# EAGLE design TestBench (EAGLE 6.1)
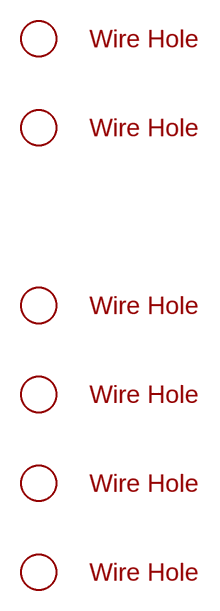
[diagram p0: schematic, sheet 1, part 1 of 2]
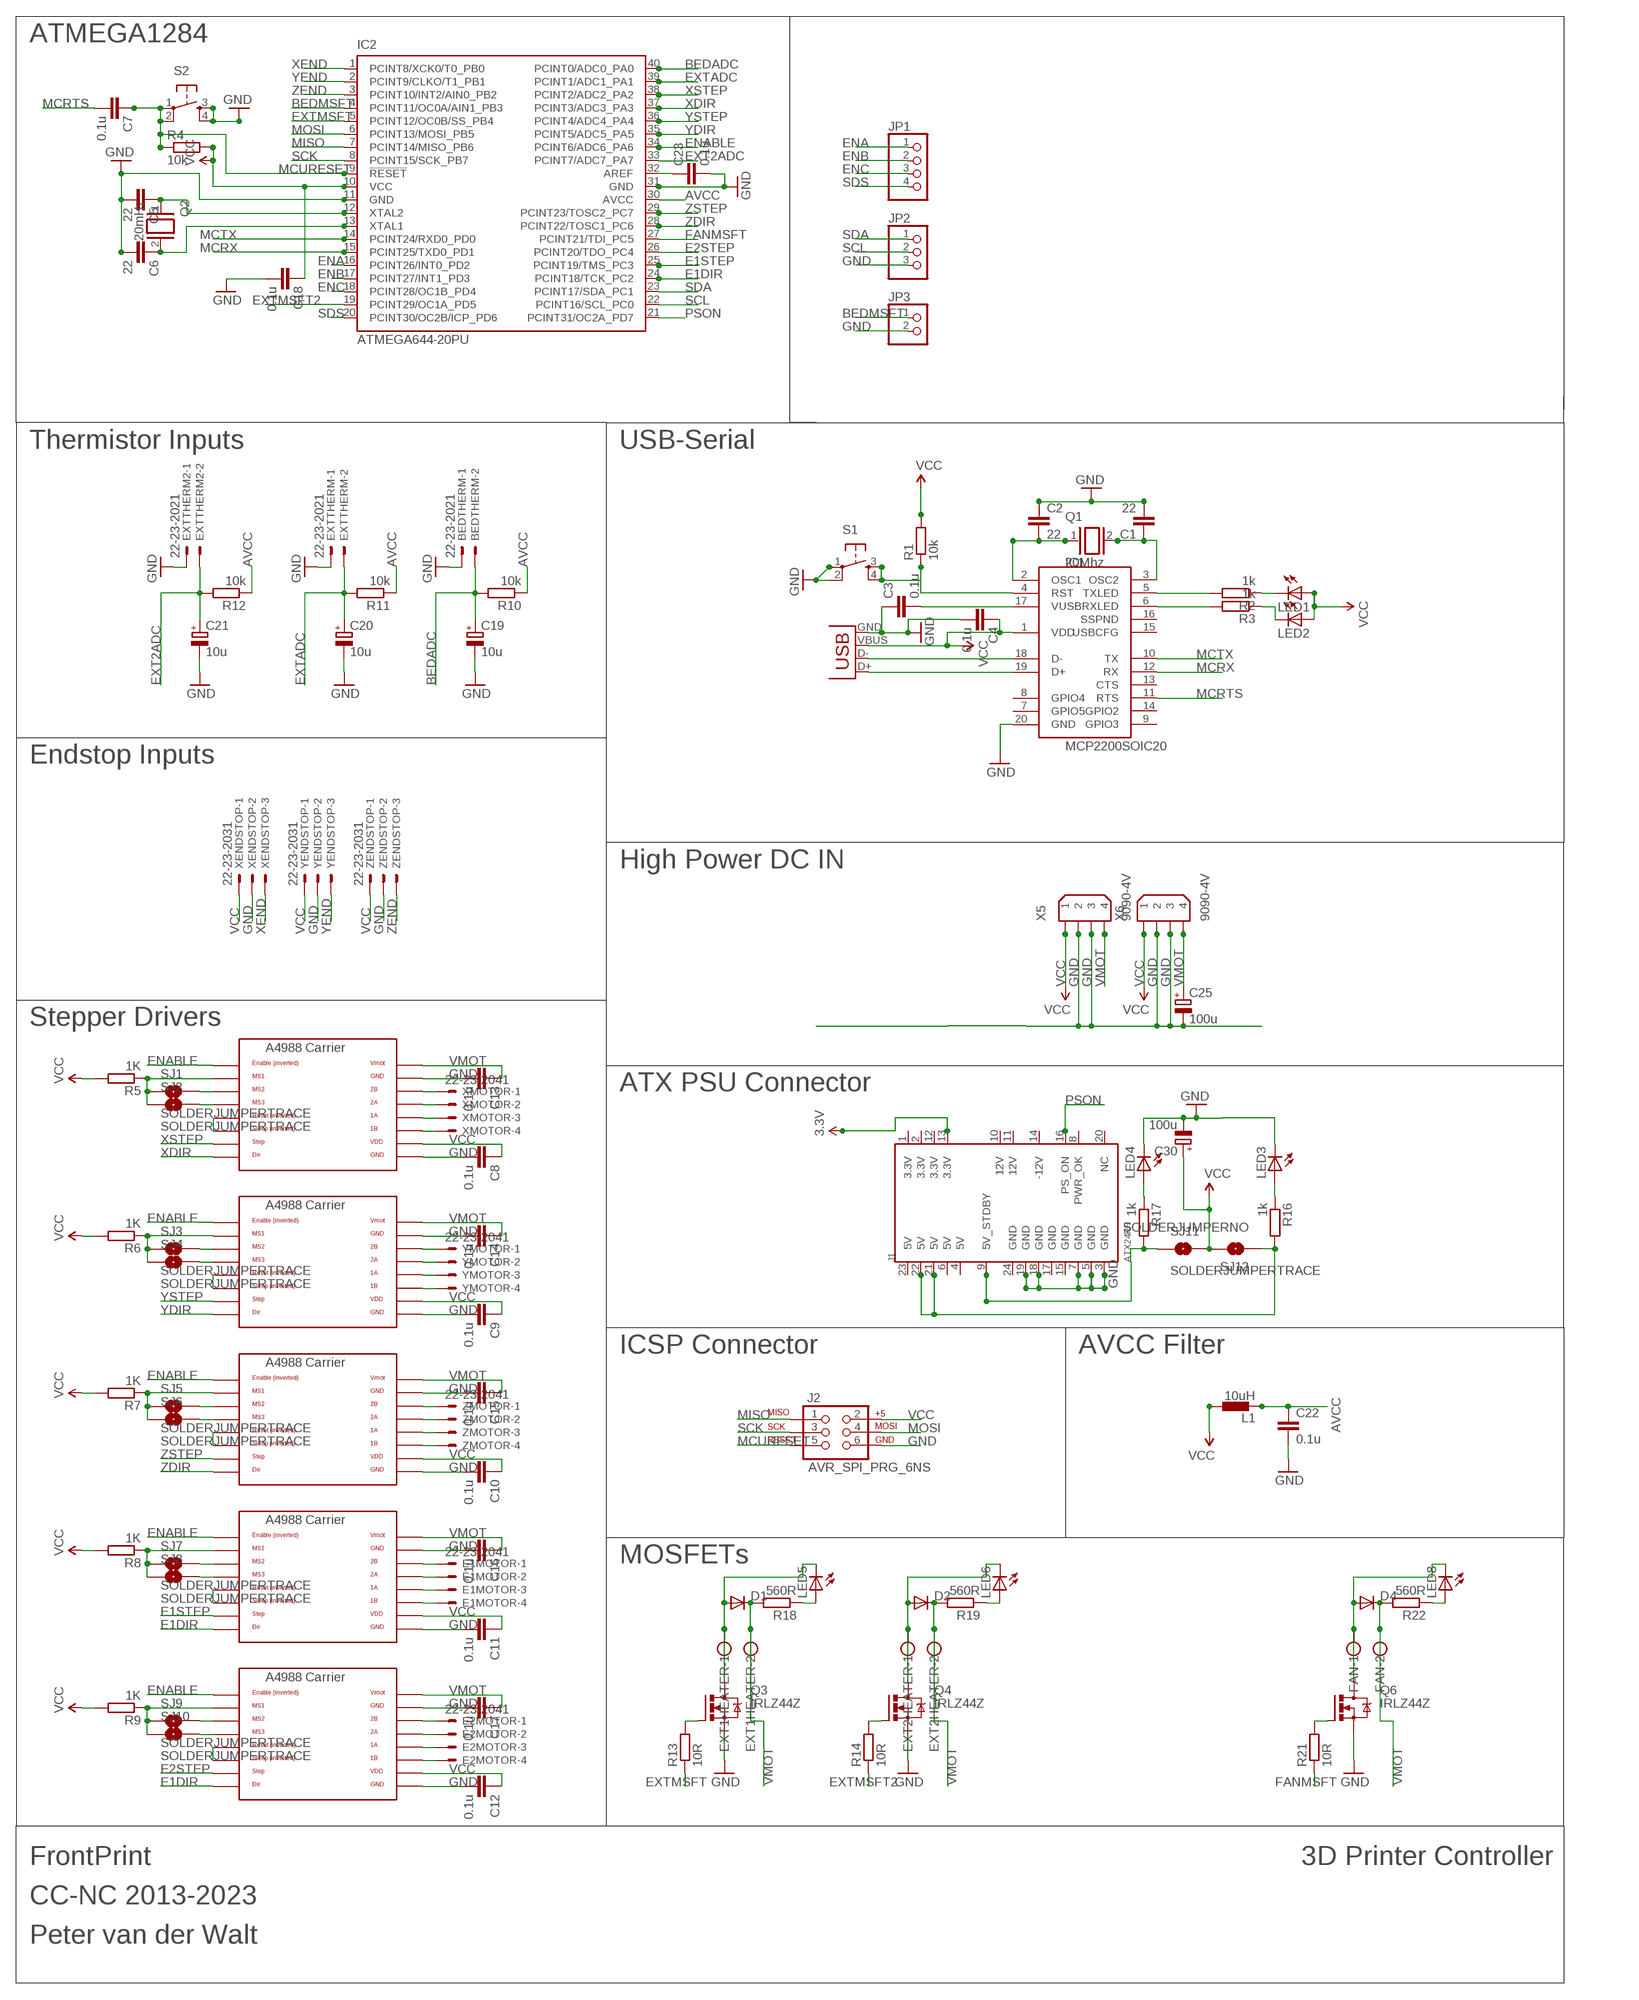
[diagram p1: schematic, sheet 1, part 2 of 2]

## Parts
BEDTHERM  22-23-2021  [22-23-2021]
C1  22  CAPKIT  [CAP-PTH-SMALL-KIT]
C2  22  CAPKIT  [CAP-PTH-SMALL-KIT]
C3  0.1u  CAPKIT  [CAP-PTH-SMALL-KIT]
C4  0.1u  CAPKIT  [CAP-PTH-SMALL-KIT]
C5  22  CAPKIT  [CAP-PTH-SMALL-KIT]
C6  22  CAPKIT  [CAP-PTH-SMALL-KIT]
C7  0.1u  CAPKIT  [CAP-PTH-SMALL-KIT]
C8  0.1u  CAPKIT  [CAP-PTH-SMALL-KIT]
C9  0.1u  CAPKIT  [CAP-PTH-SMALL-KIT]
C10  0.1u  CAPKIT  [CAP-PTH-SMALL-KIT]
C11  0.1u  CAPKIT  [CAP-PTH-SMALL-KIT]
C12  0.1u  CAPKIT  [CAP-PTH-SMALL-KIT]
C13  0.1u  CAPKIT  [CAP-PTH-SMALL-KIT]
C14  0.1u  CAPKIT  [CAP-PTH-SMALL-KIT]
C15  0.1u  CAPKIT  [CAP-PTH-SMALL-KIT]
C16  0.1u  CAPKIT  [CAP-PTH-SMALL-KIT]
C17  0.1u  CAPKIT  [CAP-PTH-SMALL-KIT]
C18  0.1u  CAPKIT  [CAP-PTH-SMALL-KIT]
C19  10u  CPOL-EUE2.5-5  [E2,5-5]
C20  10u  CPOL-EUE2.5-5  [E2,5-5]
C21  10u  CPOL-EUE2.5-5  [E2,5-5]
C22  0.1u  CAPKIT  [CAP-PTH-SMALL-KIT]
C23  0.1u  CAPKIT  [CAP-PTH-SMALL-KIT]
C25  100u  CPOL-EUE5-8.5  [E5-8,5]
C30  100u  CPOL-EUE5-8.5  [E5-8,5]
D1  DIODE1N4148  [DIODE-1N4148]
D2  DIODE1N4148  [DIODE-1N4148]
D4  DIODE1N4148  [DIODE-1N4148]
E1MOTOR  22-23-2041  [22-23-2041]
E2MOTOR  22-23-2041  [22-23-2041]
EPOLOLU  POLOLU_A4983CARRIER  [A4988BREAKOUT]
EPOLOLU2  POLOLU_A4983CARRIER  [A4988BREAKOUT]
EXT1HEATER  W237-102  [W237-102]
EXT2HEATER  W237-102  [W237-102]
EXTTHERM  22-23-2021  [22-23-2021]
EXTTHERM2  22-23-2021  [22-23-2021]
FAN  W237-102  [W237-102]
IC1  MCP2200SOIC20  [SOIC20]
IC2  ATMEGA644-20PU  [DIL40]
J1  ATX24RH  [ATX24_RIGHT_ANGLE]
J2  AVR_SPI_PRG_6NS  [2X3-NS]
JP1  PINHD-1X4  [1X04]
JP2  PINHD-1X3  [1X03]
JP3  PINHD-1X2  [1X02]
L1  10uH  BL01RN1A  [BL01RN1A]
LED1  LED3MM  [LED3MM]
LED2  LED3MM  [LED3MM]
LED3  LED3MM  [LED3MM]
LED4  LED3MM  [LED3MM]
LED5  LED3MM  [LED3MM]
LED6  LED3MM  [LED3MM]
LED8  LED3MM  [LED3MM]
Q1  20Mhz  XTAL/S  [QS]
Q2  20mHz  XTAL/S  [QS]
Q3  IRLZ44Z  [TO220BH]
Q4  IRLZ44Z  [TO220BH]
Q6  IRLZ44Z  [TO220BH]
R1  10k  R-EU_0204/7  [0204/7]
R2  1k  R-EU_0204/7  [0204/7]
R3  1k  R-EU_0204/7  [0204/7]
R4  10k  R-EU_0204/7  [0204/7]
R5  1K  R-EU_0204/7  [0204/7]
R6  1K  R-EU_0204/7  [0204/7]
R7  1K  R-EU_0204/7  [0204/7]
R8  1K  R-EU_0204/7  [0204/7]
R9  1K  R-EU_0204/7  [0204/7]
R10  10k  R-EU_0204/7  [0204/7]
R11  10k  R-EU_0204/7  [0204/7]
R12  10k  R-EU_0204/7  [0204/7]
R13  10R  R-EU_0204/7  [0204/7]
R14  10R  R-EU_0204/7  [0204/7]
R16  1k  R-EU_0204/7  [0204/7]
R17  1k  R-EU_0204/7  [0204/7]
R18  560R  R-EU_0204/7  [0204/7]
R19  560R  R-EU_0204/7  [0204/7]
R21  10R  R-EU_0204/7  [0204/7]
R22  560R  R-EU_0204/7  [0204/7]
S1  TAC_SWITCHPTH  [TACTILE-PTH]
S2  TAC_SWITCHPTH  [TACTILE-PTH]
SJ1  SOLDERJUMPERTRACE  [SJ_2S-TRACE]
SJ2  SOLDERJUMPERTRACE  [SJ_2S-TRACE]
SJ3  SOLDERJUMPERTRACE  [SJ_2S-TRACE]
SJ4  SOLDERJUMPERTRACE  [SJ_2S-TRACE]
SJ5  SOLDERJUMPERTRACE  [SJ_2S-TRACE]
SJ6  SOLDERJUMPERTRACE  [SJ_2S-TRACE]
SJ7  SOLDERJUMPERTRACE  [SJ_2S-TRACE]
SJ8  SOLDERJUMPERTRACE  [SJ_2S-TRACE]
SJ9  SOLDERJUMPERTRACE  [SJ_2S-TRACE]
SJ10  SOLDERJUMPERTRACE  [SJ_2S-TRACE]
SJ11  SOLDERJUMPERTRACE  [SJ_2S-TRACE]
SJ12  SOLDERJUMPERNO  [SJ_2S-NO]
U$1  3MMHOLE  [3MMHOLE]
U$3  3MMHOLE  [3MMHOLE]
U$5  3MMHOLE  [3MMHOLE]
U$6  3MMHOLE  [3MMHOLE]
U$7  3MMHOLE  [3MMHOLE]
U$8  3MMHOLE  [3MMHOLE]
X1  USBPTH  [USB-B-PTH]
X5  9090-4V  [9090-4V]
X6  9090-4V  [9090-4V]
XENDSTOP  22-23-2031  [22-23-2031]
XMOTOR  22-23-2041  [22-23-2041]
XPOLOLU  POLOLU_A4983CARRIER  [A4988BREAKOUT]
YENDSTOP  22-23-2031  [22-23-2031]
YMOTOR  22-23-2041  [22-23-2041]
YPOLOLU  POLOLU_A4983CARRIER  [A4988BREAKOUT]
ZENDSTOP  22-23-2031  [22-23-2031]
ZMOTOR  22-23-2041  [22-23-2041]
ZPOLOLU  POLOLU_A4983CARRIER  [A4988BREAKOUT]

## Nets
3.3V: J1.13(3.3V)
AVCC: C22.1 IC2.30(AVCC) L1.1 R10.1 R11.1 R12.1
BEDADC: BEDTHERM.2 C19.+ IC2.40(PCINT0/ADC0_PA0) R10.2
BEDMSFT: IC2.4(PCINT11/OC0A/AIN1_PB3) JP3.1
E1DIR: EPOLOLU2.DIR EPOLOLU.DIR IC2.24(PCINT18/TCK_PC2)
E1STEP: EPOLOLU.STEP IC2.25(PCINT19/TMS_PC3)
E2STEP: EPOLOLU2.STEP IC2.26(PCINT20/TDO_PC4)
ENA: IC2.16(PCINT26/INT0_PD2) JP1.1
ENABLE: EPOLOLU2.EN EPOLOLU.EN IC2.34(PCINT6/ADC6_PA6) XPOLOLU.EN YPOLOLU.EN ZPOLOLU.EN
ENB: IC2.17(PCINT27/INT1_PD3) JP1.2
ENC: IC2.18(PCINT28/OC1B_PD4) JP1.3
EXT2ADC: C21.+ EXTTHERM2.2 IC2.33(PCINT7/ADC7_PA7) R12.2
EXTADC: C20.+ EXTTHERM.2 IC2.39(PCINT1/ADC1_PA1) R11.2
EXTMSFT: IC2.5(PCINT12/OC0B/SS_PB4) R13.1
EXTMSFT2: IC2.19(PCINT29/OC1A_PD5) R14.1
FANMSFT: IC2.27(PCINT21/TDI_PC5) R21.1
GND: BEDTHERM.1 C1.2 C2.1 C3.1 C4.2 C5.2 C6.2 C8.2 C9.2 C10.2 C11.2 C12.2 C13.2 C14.2 C15.2 C16.2 C17.2 C18.2 C19.- C20.- C21.- C22.2 C23.2 C25.- C30.- EPOLOLU2.GND EPOLOLU2.GND@0(GND) EPOLOLU.GND EPOLOLU.GND@0(GND) EXTTHERM2.1 EXTTHERM.1 IC1.20(GND) IC2.11(GND) IC2.31(GND) J1.3(GND) J1.5(GND) J1.7(GND) J1.18(GND) J1.19(GND) J2.6 JP2.3 JP3.2 LED3.K(C) LED4.K(C) Q3.S Q4.S Q6.S S1.1 S1.2 S2.3 S2.4 X1.GND X5.2 X5.3 X6.2 X6.3 XENDSTOP.2 XPOLOLU.GND XPOLOLU.GND@0(GND) YENDSTOP.2 YPOLOLU.GND YPOLOLU.GND@0(GND) ZENDSTOP.2 ZPOLOLU.GND ZPOLOLU.GND@0(GND)
MCRTS: C7.2 IC1.11(RTS)
MCRX: IC1.12(RX) IC2.15(PCINT25/TXD0_PD1)
MCTX: IC1.10(TX) IC2.14(PCINT24/RXD0_PD0)
MCURESET: C7.1 IC2.9(!RESET) J2.5 R4.1 S2.1 S2.2
MISO: IC2.7(PCINT14/MISO_PB6) J2.1
MOSI: IC2.6(PCINT13/MOSI_PB5) J2.4
N$1: C2.2 IC1.2(OSC1) Q1.1
N$2: C1.1 IC1.3(OSC2) Q1.2
N$3: IC1.5(TXLED) R2.2
N$4: IC1.18(D-) X1.D-
N$5: IC1.19(D+) X1.D+
N$6: IC1.6(RXLED) R3.2
N$7: C3.2 IC1.17(VUSB)
N$8: Q3.G R13.2
N$9: LED1.K(C) R2.1
N$10: LED2.K(C) R3.1
N$11: C5.1 IC2.12(XTAL2) Q2.1
N$12: C6.1 IC2.13(XTAL1) Q2.2
N$13: IC1.4(RST) R1.1 S1.3 S1.4
N$14: R7.1 SJ5.1 SJ6.1 ZPOLOLU.MS1
N$15: SJ6.2 ZPOLOLU.MS3
N$16: SJ5.2 ZPOLOLU.MS2
N$17: EPOLOLU.MS2 SJ7.2
N$18: EPOLOLU.MS3 SJ8.2
N$19: EPOLOLU.MS1 R8.1 SJ7.1 SJ8.1
N$20: SJ3.2 YPOLOLU.MS2
N$21: SJ4.2 YPOLOLU.MS3
N$22: R6.1 SJ3.1 SJ4.1 YPOLOLU.MS1
N$23: SJ1.2 XPOLOLU.MS2
N$24: SJ2.2 XPOLOLU.MS3
N$25: R5.1 SJ1.1 SJ2.1 XPOLOLU.MS1
N$26: XPOLOLU.RST XPOLOLU.SLP(SLEEP)
N$27: YPOLOLU.RST YPOLOLU.SLP(SLEEP)
N$28: ZPOLOLU.RST ZPOLOLU.SLP(SLEEP)
N$29: EPOLOLU.RST EPOLOLU.SLP(SLEEP)
N$30: E1MOTOR.1 EPOLOLU.2B
N$31: E1MOTOR.2 EPOLOLU.2A
N$32: E1MOTOR.3 EPOLOLU.1A
N$33: E1MOTOR.4 EPOLOLU.1B
N$34: ZMOTOR.4 ZPOLOLU.1B
N$35: ZMOTOR.3 ZPOLOLU.1A
N$36: ZMOTOR.2 ZPOLOLU.2A
N$37: ZMOTOR.1 ZPOLOLU.2B
N$38: YMOTOR.4 YPOLOLU.1B
N$39: YMOTOR.3 YPOLOLU.1A
N$40: YMOTOR.2 YPOLOLU.2A
N$41: YMOTOR.1 YPOLOLU.2B
N$42: XMOTOR.4 XPOLOLU.1B
N$43: XMOTOR.3 XPOLOLU.1A
N$44: XMOTOR.2 XPOLOLU.2A
N$45: XMOTOR.1 XPOLOLU.2B
N$46: EPOLOLU2.MS2 SJ9.2
N$47: EPOLOLU2.MS3 SJ10.2
N$48: EPOLOLU2.MS1 R9.1 SJ9.1 SJ10.1
N$49: EPOLOLU2.RST EPOLOLU2.SLP(SLEEP)
N$50: E2MOTOR.1 EPOLOLU2.2B
N$51: E2MOTOR.2 EPOLOLU2.2A
N$52: E2MOTOR.3 EPOLOLU2.1A
N$53: E2MOTOR.4 EPOLOLU2.1B
N$54: C23.1 IC2.32(AREF)
N$55: D1.A EXT1HEATER.1 LED5.K(C) Q3.D
N$56: Q4.G R14.2
N$57: D2.A EXT2HEATER.1 LED6.K(C) Q4.D
N$60: J1.21(5V) J1.22(5V) R16.2 SJ12.1
N$61: LED5.A R18.1
N$62: J1.9(5V_STDBY) R17.2 SJ11.1
N$63: LED4.A R17.1
N$64: LED3.A R16.1
N$65: Q6.G R21.2
N$66: LED6.A R19.1
N$67: D4.A FAN.1 LED8.K(C) Q6.D
N$69: LED8.A R22.1
PSON: IC2.21(PCINT31/OC2A_PD7) J1.16(PS_ON)
SCK: IC2.8(PCINT15/SCK_PB7) J2.3
SCL: IC2.22(PCINT16/SCL_PC0) JP2.2
SDA: IC2.23(PCINT17/SDA_PC1) JP2.1
SDS: IC2.20(PCINT30/OC2B/ICP_PD6) JP1.4
VCC: C4.1 C8.1 C9.1 C10.1 C11.1 C12.1 C18.1 C30.+ EPOLOLU2.VDD EPOLOLU.VDD IC1.1(VDD) IC2.10(VCC) J2.2 L1.2 LED1.A LED2.A R1.2 R4.2 R5.2 R6.2 R7.2 R8.2 R9.2 SJ11.2 SJ12.2 X1.VBUS X5.1 X6.1 XENDSTOP.1 XPOLOLU.VDD YENDSTOP.1 YPOLOLU.VDD ZENDSTOP.1 ZPOLOLU.VDD
VMOT: C13.1 C14.1 C15.1 C16.1 C17.1 C25.+ D1.C D2.C D4.C EPOLOLU2.VMOT EPOLOLU.VMOT EXT1HEATER.2 EXT2HEATER.2 FAN.2 R18.2 R19.2 R22.2 X5.4 X6.4 XPOLOLU.VMOT YPOLOLU.VMOT ZPOLOLU.VMOT
XDIR: IC2.37(PCINT3/ADC3_PA3) XPOLOLU.DIR
XEND: IC2.1(PCINT8/XCK0/T0_PB0) XENDSTOP.3
XSTEP: IC2.38(PCINT2/ADC2_PA2) XPOLOLU.STEP
YDIR: IC2.35(PCINT5/ADC5_PA5) YPOLOLU.DIR
YEND: IC2.2(PCINT9/CLKO/T1_PB1) YENDSTOP.3
YSTEP: IC2.36(PCINT4/ADC4_PA4) YPOLOLU.STEP
ZDIR: IC2.28(PCINT22/TOSC1_PC6) ZPOLOLU.DIR
ZEND: IC2.3(PCINT10/INT2/AIN0_PB2) ZENDSTOP.3
ZSTEP: IC2.29(PCINT23/TOSC2_PC7) ZPOLOLU.STEP
Unconnected: IC1.7(GPIO5) IC1.8(GPIO4) IC1.9(GPIO3) IC1.13(CTS) IC1.14(GPIO2) IC1.15(USBCFG) IC1.16(SSPND) J1.1(3.3V) J1.2(3.3V) J1.4(5V) J1.6(5V) J1.8(PWR_OK) J1.10(12V) J1.11(12V) J1.12(3.3V) J1.14(-12V) J1.15(GND) J1.17(GND) J1.20(NC) J1.23(5V) J1.24(GND)

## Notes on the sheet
- ATMEGA1284
- Thermistor Inputs | USB-Serial
- Endstop Inputs
- High Power DC IN
- Stepper Drivers
- ATX PSU Connector
- ICSP Connector | AVCC Filter
- MOSFETs
- FrontPrint | 3D Printer Controller
- CC-NC 2013-2023
- Peter van der Walt

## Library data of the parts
BEDTHERM EXTTHERM EXTTHERM2 = con-molex:22-23-2021: .100" (2.54mm) Center Header - 2 Pin; MF: MOLEX; MPN: 22-23-2021; OC_FARNELL: 1462926; OC_NEWARK: 25C3832
C1-C18 C22 C23 = SparkFun-Passives:CAP: Capacitor
C19-C21 C25 C30 = rcl:CPOL-EU: POLARIZED CAPACITOR, European symbol
D1 D2 D4 = SparkFun-DiscreteSemi:DIODE: Diode
E1MOTOR E2MOTOR XMOTOR YMOTOR ZMOTOR = con-molex:22-23-2041: .100" (2.54mm) Center Header - 4 Pin; MF: MOLEX; MPN: 22-23-2041; OC_FARNELL: 1462920; OC_NEWARK: 38C0355
EPOLOLU EPOLOLU2 XPOLOLU YPOLOLU ZPOLOLU = RepRapjr:POLOLU_A4983CARRIER
EXT1HEATER EXT2HEATER FAN = con-wago-500:W237-102: WAGO SCREW CLAMP; MPN: 237-102; OC_FARNELL: unknown; OC_NEWARK: 70K9898
IC1 = microchip-update-2:MCP2200: USB 2.0 to UART Protocol Converter with GPIO
IC2 = atmel:ATMEGA644-*PU: 8-bit Microcontroller with 64K Bytes In-System Programmable Flash Auto generated by make-symbol-device-package-bsdl.ulp Rev. 34 Source: http://www.atmel.com/dyn/resources/prod_documents/doc2593.pdf; MPN: ATMEGA644-20PU; OC_FARNELL: 1288340; OC_NEWARK: 23M5060
J1 = SparkFun-Connectors:ATX24: ATX24 Pin Power Supply Connector This is a good connector for connecting a computer power supply to a PCB. It's massive, but provides many amps of power at 5V and 12V. SKU: PRT-09498
J2 = SparkFun-Connectors:AVR_SPI_PRG_6: AVR ISP 6 Pin This is the reduced ISP connector for AVR programming. Common on Arduino. This footprint will take up less PCB space and can be used with a 10-pin to 6-pin adapter such as SKU: BOB-08508
JP1 = pinhead:PINHD-1X4: PIN HEADER
JP2 = pinhead:PINHD-1X3: PIN HEADER
JP3 = pinhead:PINHD-1X2: PIN HEADER
L1 = inductors:BL0: Noise Suppression Products/EMI Suppression Filters, Lead EMIFIL(R) Inductor Type
LED1-LED6 LED8 = led:LED: LED
Q1 Q2 = special:XTAL/S: CRYSTAL
Q3 Q4 Q6 = transistor-power:IRLZ44Z: N-Channel HEXFET® Power MOSFET Logic Level AUTOMOTIVE MOSFET Source: http://www.irf.com/product-info/datasheets/data/irlz44zpbf.pdf
R1-R14 R16-R19 R21 R22 = resistor:R-EU_: RESISTOR, European symbol
S1 S2 = SparkFun-Electromechanical:TAC_SWITCH: Momentary Switch Button commonly used for reset or general input. Spark Fun Electronics SKU : COM-00097
SJ1-SJ12 = SparkFun-Passives:SOLDERJUMPER: Solder Jumper
U$1 U$3 U$5-U$8 = reprap:3MMHOLE
X1 = SparkFun-Connectors:USB: USB Connectors USB-B-PTH is fully proven SKU : PRT-00139 USB-miniB is fully proven SKU : PRT-00587 USB-A-PCB is untested. USB-A-H is throughly reviewed, but untested. Spark Fun Electronics SKU : PRT-00437 USB-B-SMT is throughly reviewed, but untested. Needs silkscreen touching up. USB-A-S has not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
X5 X6 = con-thomas-betts:9090-4: Disk Drive Power four position Source: Thomas & Betts Electronic Interconnects Eiropean Edition 1998; OC_FARNELL: unknown; OC_NEWARK: unknown
XENDSTOP YENDSTOP ZENDSTOP = con-molex:22-23-2031: .100" (2.54mm) Center Header - 3 Pin; MF: MOLEX; MPN: 22-23-2031; OC_FARNELL: 1462950; OC_NEWARK: 30C0862

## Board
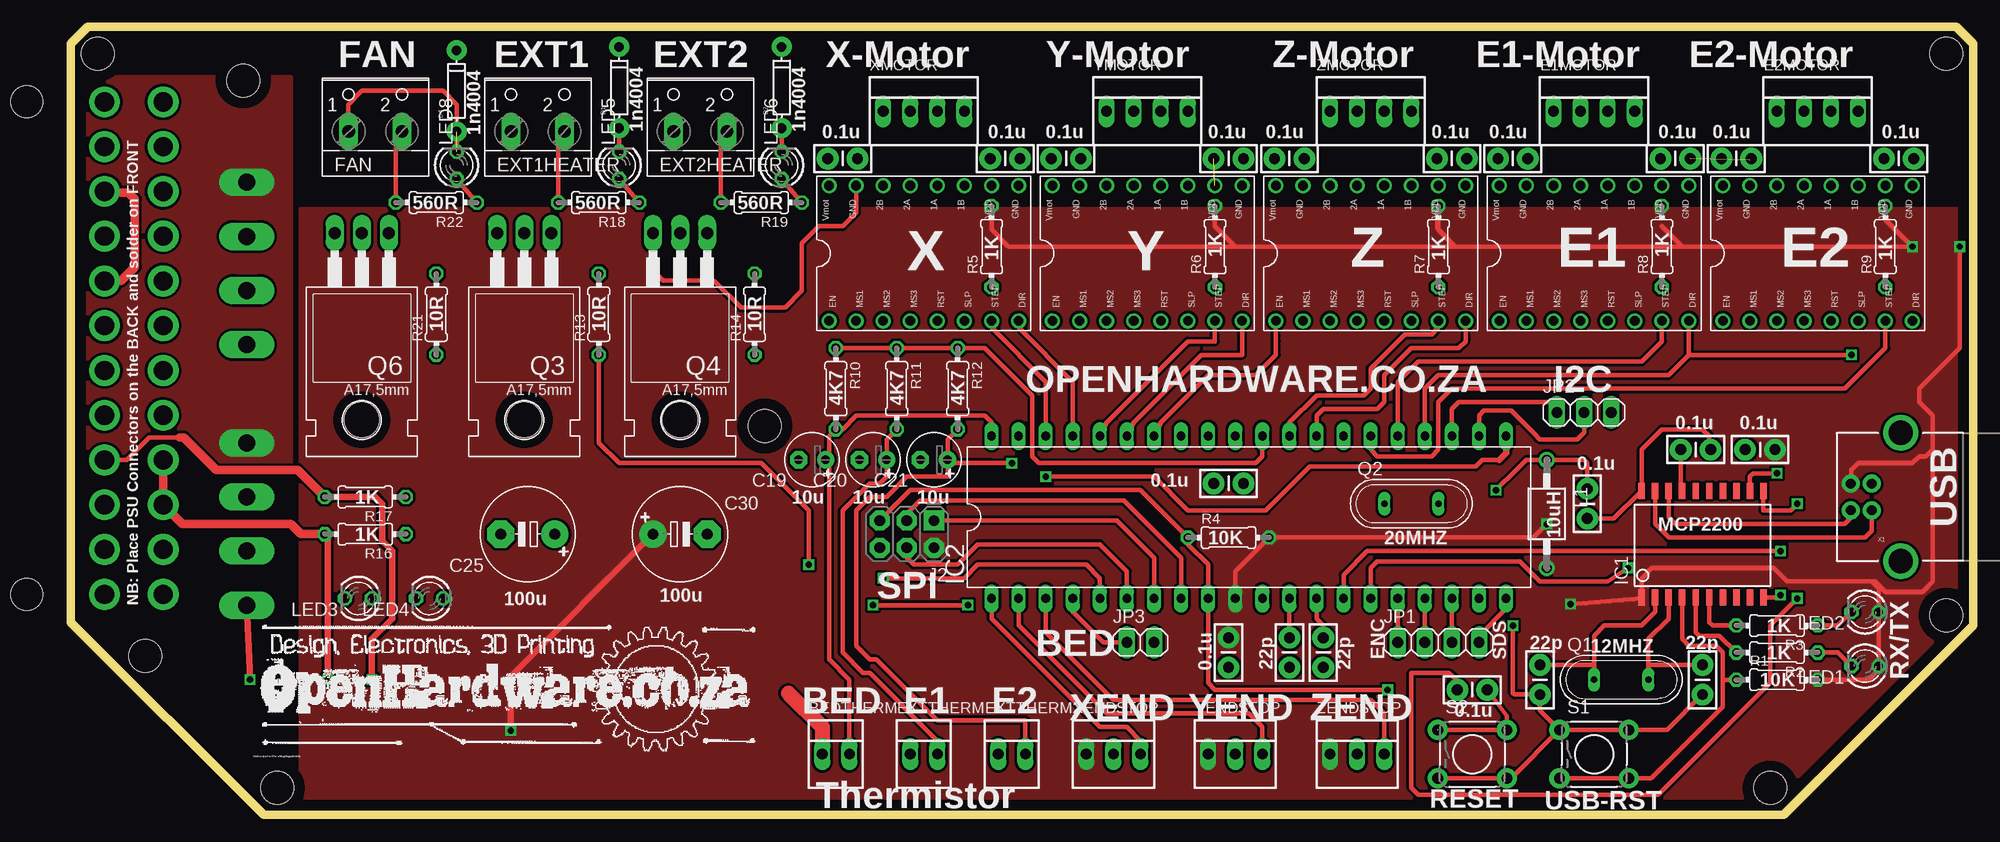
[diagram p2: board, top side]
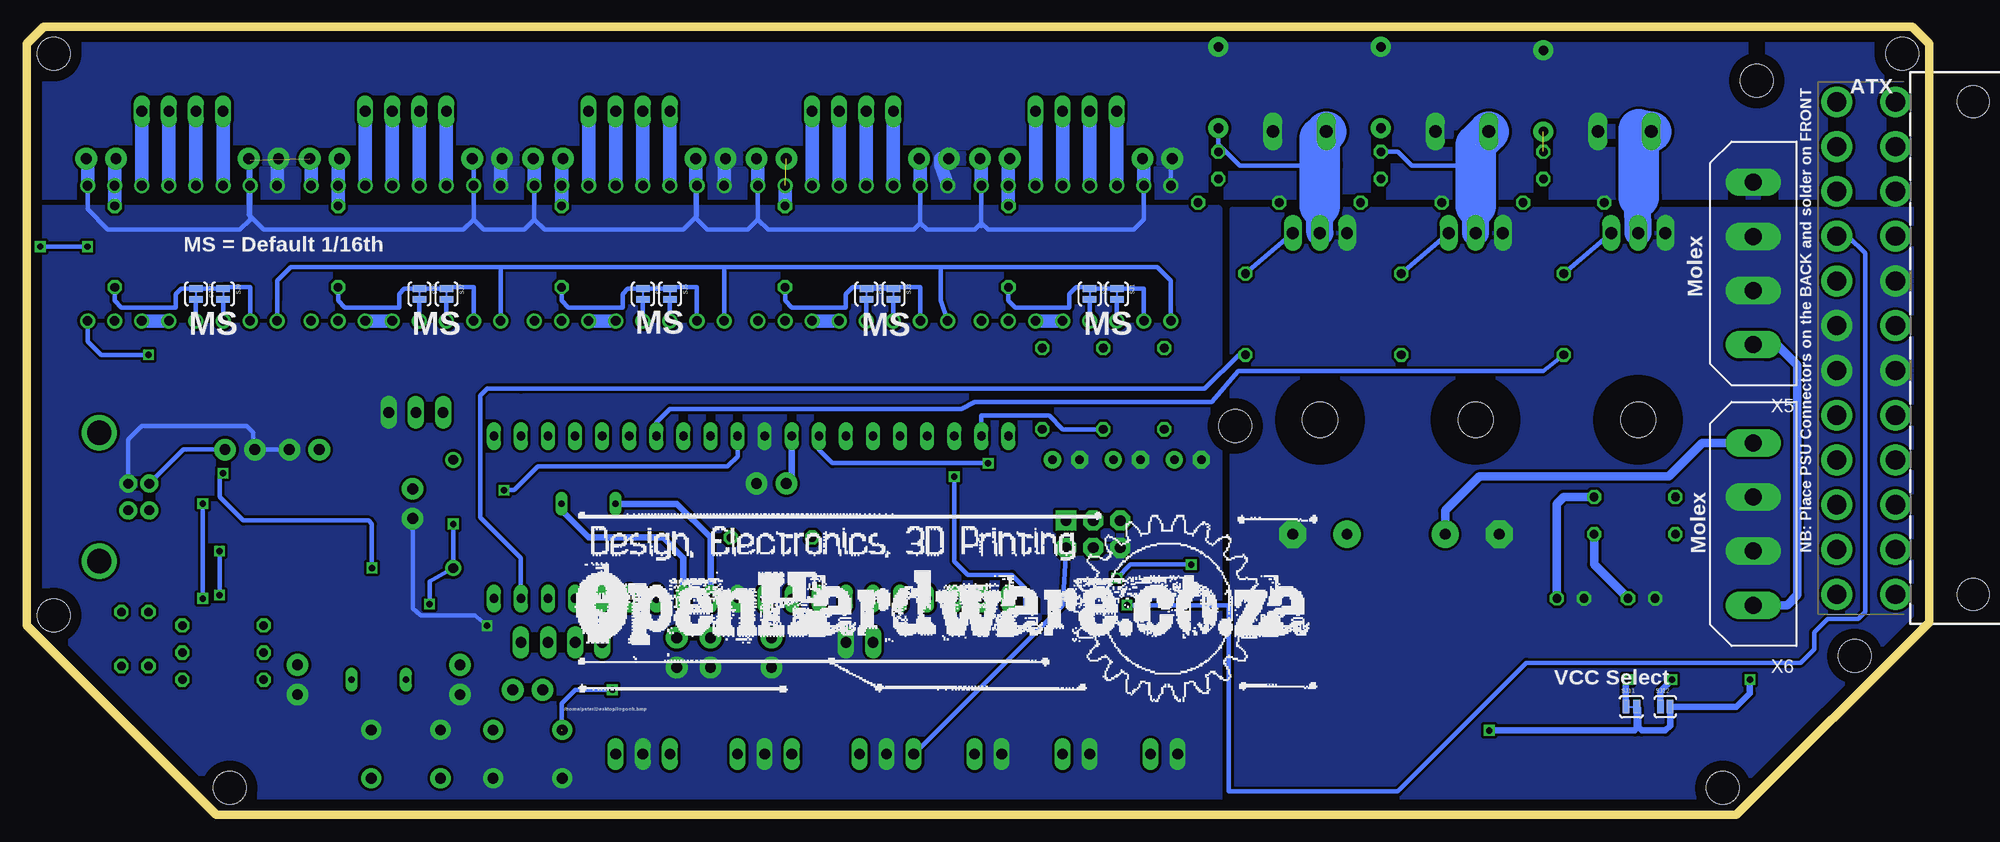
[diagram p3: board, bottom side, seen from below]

Size 178.44 x 73.98 mm. Coordinates in mm from the lower left corner, seen from the top.
Outline: 0,72.39 0,18.1 18.1,0 160.65,0 178.43,17.78 178.43,72.39 176.85,73.98 1.59,73.98 0,72.39
Copper layers (1*16): Top 0.035mm / dielectric 1.5mm / Bottom 0.035mm
Design rules: minimum track width 10mil, minimum drill 20mil, track to track 10mil, track to pad 10mil, pad to pad 10mil, via to via 10mil, smd to smd 10mil, copper to edge 40mil, drill to drill 8mil, minimum pad ring 10mil, minimum via ring 8mil, stop-mask expansion 1mil, vias tented up to drill 0mil, thermal gap 0mil

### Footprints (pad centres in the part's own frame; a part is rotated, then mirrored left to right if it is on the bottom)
22-23-2021 = drill 1 long: 1 -1.27,0; 2 1.27,0
CAP-PTH-SMALL-KIT = drill 1.016 pad 2.032: 1 -1.397,0; 2 1.397,0
E2,5-5 = drill 0.813 pad 1.6: + -1.27,0 | drill 0.813 pad 1.6 octagon: - 1.27,0
E5-8,5 = drill 1.016 pad 2.54: + -2.54,0 | drill 1.016 pad 2.54 octagon: - 2.54,0
DIODE-1N4148 = drill 0.9 pad 1.88: A -3.81,0; C 3.81,0
22-23-2041 = drill 1 long: 1 -3.81,0; 2 -1.27,0; 3 1.27,0; 4 3.81,0
A4988BREAKOUT = drill 0.9: 1A 8.89,1.27; 1B 11.43,1.27; 2A 6.35,1.27; 2B 3.81,1.27; DIR 16.51,-11.43; EN -1.27,-11.43; GND 16.51,1.27; GND@0 1.27,1.27; MS1 1.27,-11.43; MS2 3.81,-11.43; MS3 6.35,-11.43; RST 8.89,-11.43; SLP 11.43,-11.43; STEP 13.97,-11.43; VDD 13.97,1.27; VMOT -1.27,1.27
W237-102 = drill 1.194 long: 1 -2.5,-1.27; 2 2.5,-1.27
SOIC20 = smd 0.6 x 1.5: 1 -5.715,-5; 2 -4.445,-5; 3 -3.175,-5; 4 -1.905,-5; 5 -0.635,-5; 6 0.635,-5; 7 1.905,-5; 8 3.175,-5; 9 4.445,-5; 10 5.715,-5; 11 5.715,5; 12 4.445,5; 13 3.175,5; 14 1.905,5; 15 0.635,5; 16 -0.635,5; 17 -1.905,5; 18 -3.175,5; 19 -4.445,5; 20 -5.715,5
DIL40 = drill 0.813 long: 1 -24.13,-7.62; 2 -21.59,-7.62; 3 -19.05,-7.62; 4 -16.51,-7.62; 5 -13.97,-7.62; 6 -11.43,-7.62; 7 -8.89,-7.62; 8 -6.35,-7.62; 9 -3.81,-7.62; 10 -1.27,-7.62; 11 1.27,-7.62; 12 3.81,-7.62; 13 6.35,-7.62; 14 8.89,-7.62; 15 11.43,-7.62; 16 13.97,-7.62; 17 16.51,-7.62; 18 19.05,-7.62; 19 21.59,-7.62; 20 24.13,-7.62; 21 24.13,7.62; 22 21.59,7.62; 23 19.05,7.62; 24 16.51,7.62; 25 13.97,7.62; 26 11.43,7.62; 27 8.89,7.62; 28 6.35,7.62; 29 3.81,7.62; 30 1.27,7.62; 31 -1.27,7.62; 32 -3.81,7.62; 33 -6.35,7.62; 34 -8.89,7.62; 35 -11.43,7.62; 36 -13.97,7.62; 37 -16.51,7.62; 38 -19.05,7.62; 39 -21.59,7.62; 40 -24.13,7.62
ATX24_RIGHT_ANGLE = drill 1.8 pad 2.9: 1 23.1,4.76; 2 18.9,4.76; 3 14.7,4.76; 4 10.5,4.76; 5 6.3,4.76; 6 2.1,4.76; 7 -2.1,4.76; 8 -6.3,4.76; 9 -10.5,4.76; 10 -14.7,4.76; 11 -18.9,4.76; 12 -23.1,4.76; 13 23.1,10.26; 14 18.9,10.26; 15 14.7,10.26; 16 10.5,10.26; 17 6.3,10.26; 18 2.1,10.26; 19 -2.1,10.26; 20 -6.3,10.26; 21 -10.5,10.26; 22 -14.7,10.26; 23 -18.9,10.26; 24 -23.1,10.26 | hole 3: -23.1,-2.54; 23.1,-2.54
2X3-NS = drill 1.016 pad 1.88 square: 1 -2.54,-1.27 | drill 1.016 pad 1.88 octagon: 2 -2.54,1.27; 3 0,-1.27; 4 0,1.27; 5 2.54,-1.27; 6 2.54,1.27
1X04 = drill 1.016 long: 1 -3.81,0; 2 -1.27,0; 3 1.27,0; 4 3.81,0
1X03 = drill 1.016 long: 1 -2.54,0; 2 0,0; 3 2.54,0
1X02 = drill 1.016 long: 1 -1.27,0; 2 1.27,0
BL01RN1A = drill 0.9 pad 1.5: 1 -5.08,0; 2 5.08,0
LED3MM = drill 0.813 octagon: A -1.27,0; K 1.27,0
QS = drill 0.61 long: 1 -2.54,0; 2 2.54,0
TO220BH = drill 1.118 long: D 0,-6.35; G -2.54,-6.35; S 2.54,-6.35 | hole 3.302: 0,11.176
0204/7 = drill 0.813 octagon: 1 -3.81,0; 2 3.81,0
TACTILE-PTH = drill 1.016 pad 1.88: 1 -3.251,2.261; 2 3.251,2.261; 3 -3.251,-2.261; 4 3.251,-2.261
SJ_2S-TRACE = smd 0.635 x 1.27: 1 -0.508,0; 2 0.508,0
SJ_2S-NO = smd 0.635 x 1.27: 1 -0.45,0; 2 0.45,0
3MMHOLE = hole 3.1: 0,0
USB-B-PTH = drill 0.914 pad 1.676: D+ 0,1.25; D- 1.981,1.25; GND 0,-1.25; VBUS 1.981,-1.25 | drill 2.286: S1 -2.718,-6.02; S2 -2.718,6.02
9090-4V = drill 1.6 pad 2.6 long: 1 -7.62,0; 2 -2.54,0; 3 2.54,0; 4 7.62,0
22-23-2031 = drill 1 long: 1 -2.54,0; 2 0,0; 3 2.54,0

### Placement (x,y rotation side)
BEDTHERM  71.75,5.71 0 top
C1  153.03,12.7 270 top
C2  137.79,12.7 90 top
C3  152.4,34.29 180 top
C4  158.43,34.29 180 top
C5  114.3,15.24 270 top
C6  117.47,15.24 270 top
C7  131.44,11.75 180 top
C8  108.58,61.59 0 top
C9  87.63,61.59 0 top
C10  171.45,61.59 0 top
C11  150.5,61.59 0 top
C12  129.54,61.59 0 top
C13  135.25,61.59 0 top
C14  93.34,61.59 0 top
C15  156.21,61.59 0 top
C16  114.3,61.59 0 top
C17  72.39,61.59 0 top
C18  108.58,15.24 270 top
C19  69.53,33.34 180 top
C20  75.25,33.34 180 top
C21  80.96,33.34 180 top
C22  142.24,29.21 270 top
C23  108.58,31.11 0 top
C25  42.86,26.35 180 top
C30  57.15,26.35 0 top
D1  51.44,68.26 90 top
D2  66.67,68.26 90 top
D4  36.19,67.94 90 top
E1MOTOR  142.88,66.04 0 top
E2MOTOR  163.83,66.04 0 top
EPOLOLU  135.25,57.78 0 top
EPOLOLU2  156.21,57.78 0 top
EXT1HEATER  43.81,65.4 0 top
EXT2HEATER  59.06,65.4 0 top
EXTTHERM  80.01,5.71 0 top
EXTTHERM2  88.26,5.71 0 top
FAN  28.57,65.4 0 top
IC1  153.03,25.4 0 top
IC2  110.49,27.94 0 top
J1  -1.59,43.81 90 bottom
J2  78.42,26.35 180 top
JP1  128.27,16.19 0 top
JP2  141.92,37.78 0 top
JP3  100.33,16.19 0 top
L1  138.43,28.26 270 top
LED1  168.27,13.97 180 top
LED2  168.27,19.05 180 top
LED3  26.99,20.32 180 top
LED4  33.66,20.32 180 top
LED5  51.44,60.96 90 top
LED6  66.67,60.96 90 top
LED8  36.19,60.96 90 top
Q1  145.41,12.7 0 top
Q2  125.73,29.21 0 top
Q3  42.54,48.26 180 top
Q4  57.15,48.26 180 top
Q6  27.31,48.26 180 top
R1  160.02,12.7 0 top
R2  160.02,15.24 180 top
R3  160.02,17.78 180 top
R4  108.58,26.03 0 top
R5  86.36,53.34 90 top
R6  107.31,53.34 90 top
R7  128.27,53.34 90 top
R8  149.22,53.34 90 top
R9  170.18,53.34 90 top
R10  71.75,40 270 top
R11  77.47,40 270 top
R12  83.19,40 270 top
R13  49.53,46.99 90 top
R14  64.13,46.99 90 top
R16  27.62,26.35 180 top
R17  27.62,29.84 180 top
R18  49.53,57.47 180 top
R19  64.77,57.47 180 top
R21  34.29,46.99 90 top
R22  34.29,57.47 180 top
S1  142.88,5.71 0 top
S2  131.44,5.71 0 top
SJ1  76.2,48.89 270 bottom
SJ2  78.74,48.89 270 bottom
SJ3  97.16,48.89 270 bottom
SJ4  99.69,48.89 270 bottom
SJ5  118.11,48.89 270 bottom
SJ6  120.65,48.89 270 bottom
SJ7  139.06,48.89 270 bottom
SJ8  141.6,48.89 270 bottom
SJ9  160.02,48.89 270 bottom
SJ10  162.56,48.89 270 bottom
SJ11  27.94,10.16 0 bottom
SJ12  24.76,10.16 0 bottom
U$1  16.19,68.9 0 top
U$2  3MMHOLE  [3MMHOLE]  2.54,71.44 0 top
U$3  65.09,36.51 0 top
U$4  3MMHOLE  [3MMHOLE]  19.37,2.54 0 top
U$5  159.38,2.54 0 top
U$6  175.89,18.73 0 top
U$7  6.98,14.92 0 top
U$8  175.89,71.44 0 top
X1  168.91,29.84 180 top
X5  16.51,51.75 90 bottom
X6  16.51,27.3 90 bottom
XENDSTOP  97.79,5.71 0 top
XMOTOR  80.01,66.04 0 top
XPOLOLU  72.39,57.78 0 top
YENDSTOP  109.22,5.71 0 top
YMOTOR  100.97,66.04 0 top
YPOLOLU  93.34,57.78 0 top
ZENDSTOP  120.65,5.71 0 top
ZMOTOR  121.92,66.04 0 top
ZPOLOLU  114.3,57.78 0 top

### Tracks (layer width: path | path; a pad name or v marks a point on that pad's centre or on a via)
AVCC  (via drill 0.6)
  Top 0.406: IC2.30 111.76,33.65 111.12,33.02 90.8,33.02 90.17,33.65 90.17,39.37 85.72,43.81 R12.1 R11.1 R10.1 | v133.67,30.48 135.57,32.38 136.52,33.34 L1.1 141.92,33.34 142.24,33.02 C22.1
  Bottom 0.406: v133.67,30.48 132.71,30.48 130.49,32.7 112.71,32.7 111.76,33.65 IC2.30
BEDADC
  Top 0.406: IC2.40 86.36,36.83 85.72,37.46 73.66,37.46 72.39,36.19 R10.2 71.12,35.56 71.12,33.34 | BEDTHERM.2 73.02,12.7 71.12,14.6 71.12,29.84 71.12,33.34 | 71.12,33.34 C19.+
BEDMSFT
  Top 0.406: IC2.4 93.98,19.05 96.84,16.19 98.74,16.19 JP3.1
E1DIR  (via drill 0.6)
  Top 0.406: IC2.24 127,40 128.27,41.27 149.86,41.27 151.76,43.18 | 151.76,43.18 EPOLOLU.DIR 151.76,43.18 | 151.76,43.18 v167,43.18
  Bottom 0.406: v167,43.18 171.45,43.18 172.72,44.45 EPOLOLU2.DIR
E1STEP
  Top 0.406: IC2.25 124.46,40.64 126.36,42.54 147.32,42.54 149.22,44.45 EPOLOLU.STEP
E2STEP
  Top 0.406: IC2.26 121.92,34.29 122.55,33.65 127.63,33.65 128.27,34.29 128.27,38.73 129.54,40 166.37,40 170.18,43.81 EPOLOLU2.STEP
ENA
  Top 0.406: JP1.1 IC2.16
ENABLE
  Top 0.406: IC2.34 102.23,36.83 106.68,41.27 110.49,41.27 111.12,41.27 113.03,43.18 113.03,44.45 ZPOLOLU.EN
  Bottom 0.406: EPOLOLU.EN 133.98,48.26 133.98,51.43 | EPOLOLU2.EN 154.94,48.26 154.94,50.16 153.67,51.43 133.98,51.43 | 113.03,48.26 ZPOLOLU.EN 113.03,51.43 | YPOLOLU.EN 92.71,48.26 92.71,51.43 | 71.12,47.62 XPOLOLU.EN 71.12,50.16 72.39,51.43 92.71,51.43 | 92.71,51.43 113.03,51.43 | 113.03,51.43 133.98,51.43
ENB
  Top 0.406: JP1.2 IC2.17
ENC
  Top 0.406: JP1.3 IC2.18
EXT2ADC  (via drill 0.6)
  Top 0.406: v88.26,33.02 86.36,33.02 82.55,33.02 C21.+ | EXTTHERM2.2 89.53,8.89 81.28,8.89 75.56,14.6 74.93,14.6 73.66,15.87 73.66,28.57 74.93,29.84 76.52,29.84 78.42,31.75 80.01,31.75 82.23,31.75 C21.+ | C21.+ 82.23,35.24 R12.2
  Bottom 0.406: v88.26,33.02 102.87,33.02 104.14,34.29 IC2.33
EXTADC
  Top 0.406: EXTTHERM.2 81.28,6.98 74.93,13.33 74.29,13.33 72.39,15.24 72.39,28.57 74.93,31.11 75.88,31.11 76.52,31.75 C20.+ 76.52,35.24 R11.2
  Bottom 0.406: R11.2 81.28,36.19 82.55,37.46 83.18,37.46 88.9,37.46 IC2.39
EXTMSFT  (via drill 0.6)
  Top 0.406: R13.1 49.53,34.92 51.43,33.02 64.77,33.02 69.21,28.57 v69.21,23.49 | v76.2,22.22 83.82,22.22 85.09,23.49 95.25,23.49 96.52,22.22 IC2.5
  Bottom 0.406: v69.21,23.49 74.93,23.49 v76.2,22.22
EXTMSFT2
  Bottom 0.406: R14.1 64.77,43.18 67.94,40 132.08,40 135.25,40 135.89,39.37 135.89,36.83 135.89,27.94 132.08,24.13 IC2.19
FANMSFT
  Bottom 0.406: IC2.27 119.38,36.83 118.11,38.1 90.8,38.1 89.53,38.73 67.31,38.73 64.8,41.66 36.23,41.66 R21.1
GND  (via drill 0.6)  (1 unrouted)
  Top 0.406: S1.1 137.79,9.8 C2.1 135.38,11.3 135.25,11.43 135.25,16.19 v135.25,17.78 | S1.1 S1.2 149.71,7.98 C1.2 | S1.1 135.1,3.45 S2.4 S2.3 | C22.2 144.73,27.81 IC1.20 147.32,34.29 149.22,36.19 153.03,36.19 153.67,35.56 153.67,34.42 C3.1 | Q4.S 54.61,51.12 55.56,50.16 60.32,50.16 62.86,47.62 66.99,47.62 68.58,49.21 68.58,53.66 70.17,55.24 72.39,55.24 73.66,56.51 XPOLOLU.GND@0
  Top 0.813: J1.5 4.71,50.11 6.03,51.43 6.03,57.78 5.4,58.42 3.27,58.42 J1.3
  Top 1.422: 67.31,11.43 70.48,8.25 BEDTHERM.1 | BEDTHERM.1 70.48,5.4 BEDTHERM.1
  Bottom 0.406: 151.76,61.59 151.76,62.23 | X1.GND 168.91,35.24 167.64,36.51 157.8,36.51 157.16,35.88 157.16,34.42 C4.2 C3.1 | C22.2 142.21,19.4 141.48,18.73 136.4,18.73 v135.25,17.78 | 172.72,61.59 172.72,56.83 170.81,54.93 158.43,54.93 157.48,55.88 EPOLOLU2.GND@0 157.48,61.47 C15.2 157.61,56.32 156.21,54.93 137.48,54.93 136.52,55.88 | 136.52,55.88 EPOLOLU.GND@0 136.52,61.47 | 136.52,61.47 C13.2 | 136.52,61.47 136.52,55.88 | 136.52,55.88 135.57,54.93 131.76,54.93 130.81,55.88 | 130.81,55.88 ZPOLOLU.GND | 130.81,61.59 130.81,55.88 | 130.81,55.88 129.86,54.93 116.84,54.93 115.57,56.2 ZPOLOLU.GND@0 | C16.2 115.7,56.01 114.62,54.93 110.81,54.93 109.85,55.88 | 109.85,55.88 YPOLOLU.GND | 109.85,61.59 109.85,55.88 | 109.85,55.88 108.9,54.93 95.25,54.93 94.61,55.56 | 94.61,55.56 YPOLOLU.GND@0 | 88.9,55.56 88.9,61.59 88.9,55.24 | 88.9,55.56 89.53,54.93 93.98,54.93 94.61,55.56 | XPOLOLU.GND@0 73.66,55.88 74.61,54.93 88.26,54.93 88.9,55.56
  Bottom 1.27: C9.2 88.9,61.59 XPOLOLU.GND | C8.2 109.85,61.59 YPOLOLU.GND | C14.2 94.61,61.59 YPOLOLU.GND@0 | C12.2 130.81,61.59 ZPOLOLU.GND | C11.2 151.76,61.59 EPOLOLU.GND | C10.2 172.72,61.59 EPOLOLU2.GND | C17.2 73.66,61.59 XPOLOLU.GND@0 | ZPOLOLU.GND@0 115.7,59.05 C16.2
  pour Bottom: 177.48,56.83 66.67,56.83 66.67,1.27 160.02,1.27 177.48,18.73
  pour Bottom: 0.63,56.83 65.41,56.83 65.41,0.95 18.41,0.95 0.63,18.73
MCRTS  (via drill 0.6)
  Top 0.406: IC1.11 158.75,28.57 161.29,28.57 v161.92,29.21 | v161.92,20.32 159.38,17.78 159.38,12.38 148.91,1.9 126.36,1.9 125.73,2.54 125.73,13.33 129.22,13.33 129.98,12.7 C7.2
  Bottom 0.406: v161.92,29.21 v161.92,20.32
MCRX  (via drill 0.6)
  Top 0.406: IC2.15 121.92,23.18 122.55,23.81 135.89,23.81 137.79,21.91 144.14,21.91 v146.05,23.18 | v160.02,32.07 157.8,32.07 157.48,31.75 IC1.12
  Bottom 0.406: v146.05,23.18 146.05,27.3 146.37,27.62 158.11,27.62 160.34,29.84 160.34,31.75 v160.02,32.07
MCTX  (via drill 0.6)
  Top 0.406: IC1.10 160.1,20.4 v160.34,20.64 | v160.34,24.76 121.6,24.76 119.38,22.54 IC2.14
  Bottom 0.406: v160.34,20.64 v160.34,24.76
MCURESET  (via drill 0.6)  (1 unrouted)
  Top 0.406: J2.5 78.74,30.48 100.33,30.48 R4.1 104.77,25.4 106.68,23.49 IC2.9 106.68,12.38 107.31,11.75 v123.51,11.75 | S2.1 S2.2 134.7,9.32 C7.1
  Bottom 0.406: v123.51,11.75 127,11.75 128.27,10.48 128.27,7.94
MISO
  Top 0.406: IC2.7 101.6,24.13 98.11,27.62 J2.1
MOSI
  Top 0.406: IC2.6 99.06,22.86 96.52,25.4 85.09,25.4 83.18,23.49 79.06,23.49 78.42,24.13 J2.4
N$1
  Top 0.406: IC1.2 148.59,19.05 147.32,17.78 143.83,17.78 142.87,16.83 142.87,14.29 | 142.87,14.29 Q1.1 | C2.2 142.68,14.1 142.87,14.29
N$2
  Top 0.406: IC1.3 149.86,18.41 147.95,16.51 147.95,13.97 | 147.95,13.97 Q1.2 | C1.1 148.08,14.1 147.95,13.97
N$3
  Top 0.406: IC1.5 152.4,17.14 152.72,16.83 154.62,16.83 R2.2
N$4
  Top 0.406: IC1.18 149.86,27.94 150.49,27.3 166.37,27.3 167,27.94 167,28.52 X1.D-
N$5
  Top 0.406: IC1.19 148.59,27.3 149.86,26.03 168.27,26.03 168.91,26.67 X1.D+
N$6
  Top 0.406: IC1.6 153.67,18.1 153.99,17.78 R3.2
N$7
  Top 0.406: C3.2 151,30.53 IC1.17
N$8
  Bottom 0.406: Q3.G R13.2
N$9
  Top 0.406: R2.1 165.73,15.24 LED1.K
N$10
  Top 0.406: R3.1 165.73,17.78 LED2.K
N$11
  Top 0.406: C5.1 IC2.12
  Bottom 0.61: IC2.12 114.3,26.03 117.47,29.21 Q2.1
N$12
  Top 0.406: C6.1 117.47,17.78 116.84,18.41 IC2.13
  Bottom 0.61: IC2.13 116.84,24.13 118.74,26.03 125.73,26.03 128.27,28.57 Q2.2
N$13
  Top 0.406: IC1.4 151.13,16.51 151.76,15.87 154.3,15.87 154.94,15.24 154.94,13.33 154.94,12.7 | 154.94,12.7 155.57,12.7 R1.1 | S1.3 S1.4 148.23,3.45 154.94,10.16 154.94,12.38 154.94,12.7
N$14
  Bottom 0.406: ZPOLOLU.MS1 115.57,49.53 118.11,49.53 SJ5.1 SJ6.1 122.05,49.4 122.55,48.89 122.55,47.62 127.63,47.62 128.27,48.26 R7.1 128.27,49.4
N$15
  Bottom 0.406: SJ6.2 ZPOLOLU.MS3
N$16
  Bottom 0.406: SJ5.2 ZPOLOLU.MS2
N$17
  Bottom 0.406: SJ7.2 EPOLOLU.MS2
N$18
  Bottom 0.406: SJ8.2 EPOLOLU.MS3
N$19
  Bottom 0.406: EPOLOLU.MS1 136.52,49.53 139.06,49.53 SJ7.1 SJ8.1 143,49.4 143.51,48.89 143.51,47.62 148.59,47.62 149.22,48.26 R8.1 149.22,49.4
N$20
  Bottom 0.406: SJ3.2 YPOLOLU.MS2
N$21
  Bottom 0.406: SJ4.2 YPOLOLU.MS3
N$22
  Bottom 0.406: YPOLOLU.MS1 94.61,49.53 96.52,49.53 | 96.52,49.53 97.15,49.53 SJ3.1 SJ4.1 | 99.69,49.53 96.52,49.53 | SJ4.1 99.69,49.53 | SJ4.1 99.69,49.53 | 99.69,49.53 100.96,49.53 101.6,48.89 101.6,47.62 106.68,47.62 107.31,48.26 R6.1
N$23
  Bottom 0.406: SJ1.2 XPOLOLU.MS2
N$24
  Bottom 0.406: SJ2.2 XPOLOLU.MS3
N$25
  Bottom 0.406: XPOLOLU.MS1 73.66,49.4 SJ1.1 SJ2.1 78.74,49.53 80.01,49.53 80.64,48.89 80.64,47.62 85.72,47.62 86.36,48.26 R5.1
N$26
  Bottom 1.27: XPOLOLU.SLP XPOLOLU.RST
N$27
  Bottom 1.27: YPOLOLU.RST YPOLOLU.SLP
N$28
  Bottom 1.27: ZPOLOLU.RST ZPOLOLU.SLP
N$29
  Bottom 1.27: EPOLOLU.RST EPOLOLU.SLP
N$30
  Bottom 1.27: E1MOTOR.1 EPOLOLU.2B
N$31
  Bottom 1.27: E1MOTOR.2 EPOLOLU.2A
N$32
  Bottom 1.27: E1MOTOR.3 EPOLOLU.1A
N$33
  Bottom 1.27: E1MOTOR.4 EPOLOLU.1B
N$34
  Bottom 1.27: ZMOTOR.4 ZPOLOLU.1B
N$35
  Bottom 1.27: ZMOTOR.3 ZPOLOLU.1A
N$36
  Bottom 1.27: ZMOTOR.2 ZPOLOLU.2A
N$37
  Bottom 1.27: ZMOTOR.1 118.11,59.69 ZPOLOLU.2B
N$38
  Bottom 1.27: YMOTOR.4 YPOLOLU.1B
N$39
  Bottom 1.27: YMOTOR.3 YPOLOLU.1A
N$40
  Bottom 1.27: YMOTOR.2 YPOLOLU.2A
N$41
  Bottom 1.27: YMOTOR.1 97.15,59.69 YPOLOLU.2B
N$42
  Bottom 1.27: XMOTOR.4 XPOLOLU.1B
N$43
  Bottom 1.27: XMOTOR.3 XPOLOLU.1A
N$44
  Bottom 1.27: XMOTOR.2 XPOLOLU.2A
N$45
  Bottom 1.27: XMOTOR.1 XPOLOLU.2B
N$46
  Bottom 0.406: SJ9.2 EPOLOLU2.MS2
N$47
  Bottom 0.406: SJ10.2 EPOLOLU2.MS3
N$48
  Bottom 0.406: EPOLOLU2.MS1 157.48,49.53 160.02,49.53 SJ9.1 SJ10.1 163.96,49.4 164.46,48.89 164.46,47.62 169.54,47.62 170.18,48.26 R9.1 170.18,49.4
N$49
  Bottom 1.27: EPOLOLU2.RST EPOLOLU2.SLP
N$50
  Bottom 1.27: E2MOTOR.1 EPOLOLU2.2B
N$51
  Bottom 1.27: E2MOTOR.2 162.56,59.69 EPOLOLU2.2A
N$52
  Bottom 1.27: E2MOTOR.3 EPOLOLU2.1A
N$53
  Bottom 1.27: E2MOTOR.4 EPOLOLU2.1B
N$54
  Bottom 0.61: IC2.32 106.68,31.56 C23.1
N$55  (1 unrouted)
  Top 0.406: LED5.K D1.A
  Bottom 0.406: LED5.K 49.85,62.23 48.53,60.92 43.2,60.92 43.2,62.22 42.53,62.88
  Bottom 2.54: Q3.D 42.54,55.88 42.54,57.15
  Bottom 3.81: 42.54,57.15 42.54,62.9 EXT1HEATER.1
N$56
  Bottom 0.406: Q4.G R14.2
N$57
  Top 0.406: LED6.K D2.A
  Bottom 0.406: D2.A 66.67,62.96 64.66,60.95 57.21,60.95 57.15,61.01
  Bottom 2.54: Q4.D 57.15,55.88 57.15,57.15
  Bottom 3.81: 57.15,57.15 57.15,61.01 57.15,63.54 EXT2HEATER.1
N$60  (via drill 0.6)
  Top 0.406: J1.22 8.67,28.99 8.89,28.89 | 24.26,25.9 R16.2
  Top 0.61: v24.13,12.7 24.13,26.03 R16.2
  Top 0.813: J1.21 J1.22 10.48,27.3 20.64,27.3 21.59,26.35 R16.2
  Bottom 0.61: SJ12.1 25.21,11.61 v24.13,12.7
N$61
  Top 0.406: LED5.A R18.1
N$62  (via drill 0.6)
  Top 0.406: J1.9 5.26,33.31 7.38,35.44 10.21,35.44
  Top 0.61: v28.26,12.7 28.26,16.51 30.16,18.41 30.16,24.76 29.21,25.72 29.21,29.21 28.57,29.84 R17.2
  Top 0.813: 10.21,35.44 10.6,35.44 13.65,32.38 21.27,32.38 R17.2
  Bottom 0.61: SJ11.1 28.45,12.51 v28.26,12.7
N$63
  Bottom 0.813: R17.1 34.29,29.84 34.92,29.21 LED4.A
N$64
  Bottom 0.813: R16.1 31.43,23.49 LED3.A
N$65
  Bottom 0.406: Q6.G R21.2
N$66
  Top 0.406: LED6.A R19.1
N$67  (1 unrouted)
  Top 0.406: LED8.K 36.19,66.67 34.92,67.94 27.3,67.94 26.03,66.67 26.03,64.17 FAN.1
  Bottom 2.54: Q6.D 27.34,57.4 27.24,57.94
  Bottom 3.81: 27.24,57.94 27.24,64.33 FAN.1
N$69
  Top 0.406: LED8.A R22.1
PSON  (via drill 0.6)
  Top 0.406: 133.98,33.34 132.4,33.34 131.76,32.7 116.2,32.7 112.08,28.57 104.77,28.57 101.6,31.75 v91.44,31.75 | v84.14,19.68 v75.25,19.68
  Top 0.61: IC2.21 134.62,33.97 133.98,33.34
  Bottom 0.406: v91.44,31.75 91.44,23.81 90.17,22.54 86.04,22.54 84.77,21.27 84.77,19.68 v84.14,19.68 | v75.25,19.68 65.72,19.68 65.72,2.22 51.12,2.22 49.85,2.22 37.78,14.29 12.06,14.29 10.79,15.56 10.79,17.14 9.52,18.41 6.67,18.41 6.03,19.05 6.03,52.7 7.62,54.29 8.57,54.29 | 8.57,54.29 8.89,54.29 | J1.16 8.59,54.31 8.57,54.29
SCK
  Top 0.406: J2.3 78.42,28.26 79.69,29.53 98.74,29.53 104.14,24.13 IC2.8
SCL
  Top 0.406: IC2.22 132.08,37.46 132.52,37.97 135.1,37.94 137.16,35.88 137.79,35.24 141.29,35.24 141.92,35.88 JP2.2
SDA
  Top 0.406: IC2.23 129.54,38.1 130.17,38.73 139.06,38.73 139.38,38.42 JP2.1
SDS
  Top 0.406: JP1.4 132.08,16.83 134.62,19.37 IC2.20
VCC  (via drill 0.6)  (1 unrouted)
  Top 0.406: R9.2 170.18,55.88 v172.72,53.34 151.13,53.34 | v177.16,53.34 177.16,43.81 173.35,40 173.35,38.73 174.62,37.46 174.62,34.29 | 174.62,34.29 173.99,33.65 173.35,33.65 172.72,33.02 167.64,33.02 167,32.38 167,31.11 166.95,31.11 X1.VBUS | R1.2 168.59,12.7 169.54,13.65 LED1.A LED2.A 169.54,21.27 168.91,21.91 | 168.91,21.91 160.97,21.91 159.7,23.18 148.27,23.18 147.32,22.22 147.32,20.32 | 147.32,20.32 IC1.1 | 168.91,21.91 169.23,21.91 170.18,20.95 173.67,20.95 174.62,21.91 174.62,34.29 | IC2.10 109.22,22.86 R4.2 137.16,26.03 v138.43,27.3 | v140.65,19.78 147.32,20.32 | 149.22,55.24 151.13,53.34 | R7.2 128.27,54.93 129.86,53.34 | 129.86,53.34 151.13,53.34 | 128.14,57.28 128.14,55.05 129.86,53.34 | 129.86,53.34 109.22,53.34 | 109.22,53.34 107.31,55.24 | 107.31,55.24 R6.2 107.31,55.24 | 107.31,55.24 109.22,53.34 | 109.22,53.34 87.95,53.34 86.36,54.93 R5.2
  Top 0.61: v16.83,12.7 X6.1 | v41.27,7.94 41.27,13.02 C30.+
  Bottom 0.406: C10.1 170.05,57.28 R9.2 | C11.1 149.1,57.28 R8.2 | C12.1 128.14,57.28 R7.2 | J2.2 81.28,19.68 XENDSTOP.1 | v172.72,53.34 176.53,53.34 v177.16,53.34 | C4.1 163.73,34.29 X1.VBUS | v138.43,27.3 L1.2 140.65,21.91 v140.65,19.78
  Bottom 0.61: v16.83,12.7 16.83,11.43 18.1,10.16 SJ12.2 24.31,8.39 24.76,7.94 26.99,7.94 27.3,8.25 27.3,10.03 SJ11.2 27.43,8.13 27.62,7.94 v41.27,7.94
  Bottom 0.813: X6.1 13.33,19.68 12.38,20.64 12.38,42.23 14.29,44.13 X5.1
  Bottom 1.27: C9.1 86.36,61.59 XPOLOLU.VDD R5.2 | C12.1 128.27,61.59 ZPOLOLU.VDD R7.2 | C11.1 149.22,61.59 EPOLOLU.VDD R8.2 | C10.1 170.18,61.59 EPOLOLU2.VDD R9.2 | YPOLOLU.VDD R6.2
  pour Top: 21.59,0.63 160.34,0.95 177.8,18.41 177.8,56.83 21.59,56.83
VMOT
  Top 0.406: R22.2 30.48,62.23 30.48,64.13 FAN.2 | R18.2 45.72,62.23 45.72,64.13 EXT1HEATER.2 | R19.2 60.96,63.5 60.96,64.13 EXT2HEATER.2
  Bottom 0.406: C13.1 133.86,62.36 | C15.1 154.81,61.72 | XPOLOLU.VMOT 71.12,61.47 C17.1
  Bottom 0.813: X6.4 21.27,34.92 24.45,31.75 42.23,31.75 45.4,28.57 C25.+
  Bottom 1.27: 154.94,61.59 C15.1 154.94,61.47 EPOLOLU2.VMOT | 113.03,61.59 C16.1 113.03,61.47 ZPOLOLU.VMOT | EPOLOLU.VMOT 133.98,61.47 C13.1 | YPOLOLU.VMOT 92.71,60.96 92.71,61.59 C14.1
  pour Bottom: 0.95,58.42 177.17,58.42 177.17,73.02 0.95,73.02
  pour Top: 0.63,69.21 20.64,69.21 20.64,0.95 20.32,0.63 18.41,0.63 0.63,18.1
XDIR
  Top 0.406: IC2.37 93.98,40.64 88.9,45.72 XPOLOLU.DIR
XEND
  Top 0.406: XENDSTOP.3 100.33,6.98 99.06,8.25 96.52,8.25 86.36,18.41 IC2.1
XSTEP
  Top 0.406: IC2.38 91.44,40.64 86.36,45.72 XPOLOLU.STEP
YDIR
  Top 0.406: IC2.35 99.69,36.83 106.04,43.18 109.85,43.18 YPOLOLU.DIR
YEND
  Top 0.406: YENDSTOP.3 111.76,8.25 110.49,9.52 97.15,9.52 88.9,17.78 IC2.2
YSTEP
  Top 0.406: IC2.36 97.15,36.83 104.77,44.45 107.31,44.45 YPOLOLU.STEP
ZDIR
  Top 0.406: IC2.28 116.84,37.46 117.47,38.1 122.55,38.1 123.19,38.73 123.19,41.27 125.73,43.81 130.17,43.81 130.81,44.45 ZPOLOLU.DIR
ZEND
  Top 0.406: ZENDSTOP.3 123.19,9.52 121.92,10.79 97.79,10.79 91.44,17.14 IC2.3
ZSTEP
  Top 0.406: IC2.29 114.3,36.83 116.84,39.37 119.38,39.37 121.28,39.37 121.92,40 121.92,41.91 125.09,45.08 127.63,45.08 128.27,45.72 ZPOLOLU.STEP

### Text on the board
tPlace: FAN | EXT1 | EXT2 | X-Motor | Y-Motor | Z-Motor | E1-Motor | E2-Motor | 1n4004 | 1n4004 | 1n4004 | 0.1u | 0.1u | 0.1u | 0.1u | 0.1u | 0.1u | 0.1u | 0.1u | 0.1u | 0.1u | 560R | 560R | 560R | 1K | 1K | 1K | Z | 1K | E1 | E2 | 1K | X | Y | 10R | 10R | 10R | OPENHARDWARE.CO.ZA | I2C | 4K7 | 4K7 | 4K7 | 0.1u | 0.1u | 0.1u | + | + | + | 0.1u | 1K | 10u | 10u | 10u | + | MCP2200 | USB | 1K | 10K | 20MHZ | 10uH | + | SPI | NB: Place PSU Connectors on the BACK and solder on FRONT | 100u | 100u | 0.1u | 1K | 22p | 12MHZ | 22p | BED | ENC | SDS | 1K | 22p | 22p | RX/TX | 10K | 0.1u | BED | E1 | E2 | XEND | YEND | ZEND | /home/peter/Desktop/logooh.bmp | Thermistor | RESET | USB-RST
bPlace: NB: Place PSU Connectors on the BACK and solder on FRONT | ATX | Molex | MS = Default 1/16th | MS | MS | MS | MS | MS | Molex | VCC Select | /home/peter/Desktop/logooh.bmp

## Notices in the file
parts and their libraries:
SparkFun-Passives: Licensing: CC v3.0 Share-Alike You are welcome to use this library for commercial purposes.
